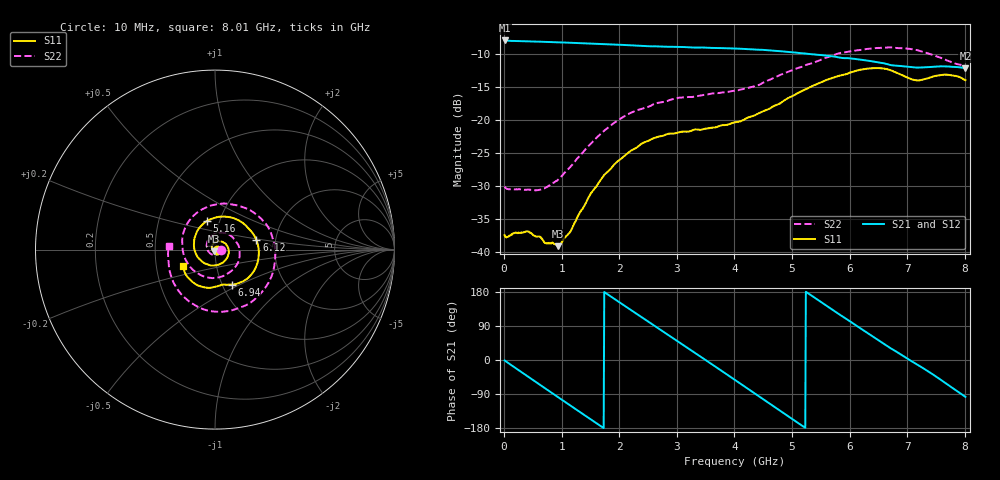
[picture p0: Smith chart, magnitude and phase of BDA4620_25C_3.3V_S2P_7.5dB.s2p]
!Agilent Technologies,E5071B,MY42404982,A.09.10
!Date: Wed May 06 08:49:57 2026
!Data & Calibration Information:
!Freq	S11:SOLT2(ON)	S21:SOLT2(ON)	S12:SOLT2(ON)	S22:SOLT2(ON)
# Hz S RI R 50
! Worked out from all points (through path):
!   801 points, 10 MHz to 8.01 GHz, reference 50 ohm
!   highest |S21| = -7.94 dB at 10 MHz (marker M1); lowest = -12.1 dB at 8.01 GHz (marker M2)
!   group delay of S21, straight-line fit = 283 ps
!   lowest |S11| = -39.1 dB at 930 MHz (marker M3), VSWR 1.02, Z = 49.4 - j0.922 ohm
!   |S11| at or under -10 dB: start of sweep to end of sweep
!   |S22| runs from -30.6 to -9.0 dB; largest |S21 - S12| = 0.0017
!   S11 on the Smith chart (normalised r, x): 10 MHz: 1.03, -0.00; 5.16 GHz: 0.87, +0.29; 6.12 GHz: 1.59, +0.18; 6.94 GHz: 1.11, -0.45; 8.01 GHz: 0.69, -0.13
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1e7  0.0135 -0.000766  0.4009 -0.00861  0.4014 -0.00861  0.0313 -0.00237
5.2e8  0.00954 -0.00939  0.2279 -0.3207  0.2281 -0.3214  0.00745 -0.0286
9.3e8  -0.00609 -0.00933  -0.0485 -0.3853  -0.049 -0.3859  -0.0302 -0.0181
1.35e9  -0.0175 0.0117  -0.2956 -0.2424  -0.2958 -0.2427  -0.0453 0.0327
1.65e9  -0.00895 0.0327  -0.373 -0.0559  -0.3734 -0.0561  -0.0225 0.0732
1.94e9  0.0128 0.0457  -0.3475 0.1346  -0.3479 0.1348  0.0249 0.0941
2.32e9  0.0497 0.0385  -0.1824 0.318  -0.1829 0.3182  0.0962 0.0707
2.68e9  0.0749 0.00533  0.0409 0.3588  0.0414 0.3593  0.1353 0.00517
3e9  0.0715 -0.0363  0.2259 0.2785  0.2263 0.2785  0.1288 -0.0706
3.39e9  0.0363 -0.0765  0.3478 0.069  0.3483 0.0683  0.0549 -0.1429
3.69e9  -0.00824 -0.0883  0.3315 -0.1179  0.3311 -0.1188  -0.0351 -0.1561
4.01e9  -0.0616 -0.0741  0.211 -0.2769  0.2108 -0.2775  -0.1292 -0.1064
4.53e9  -0.1172 0.0158  -0.0972 -0.3256  -0.098 -0.3259  -0.1813 0.0727
4.86e9  -0.1024 0.0964  -0.2569 -0.2083  -0.2573 -0.2084  -0.1119 0.1965
5.16e9  -0.045 0.1595  -0.318 -0.0456  -0.3183 -0.0455  0.0121 0.2522
5.35e9  0.0115 0.181  -0.3093 0.0612  -0.3093 0.0616  0.1013 0.2502
5.75e9  0.144 0.1557  -0.1847 0.2393  -0.1842 0.24  0.2708 0.158
6.12e9  0.231 0.0526  -0.00214 0.2898  -0.00142 0.2902  0.3362 -0.0267
6.68e9  0.1772 -0.1639  0.2186 0.147  0.2195 0.147  0.2045 -0.2903
6.94e9  0.0921 -0.1955  0.2519 0.0426  0.2526 0.0419  0.0702 -0.343
7.49e9  -0.0371 -0.213  0.187 -0.172  0.187 -0.1728  -0.2025 -0.2309
8.01e9  -0.1774 -0.0938  -0.0312 -0.2453  -0.0316 -0.2461  -0.257 0.0214
